FUNCTION "CENTR. 3  POSTERIORE DX" : VOID
TITLE =
VERSION : 0.1

BEGIN
NETWORK
TITLE =LETTURA STATUS WORD DA DRIVE
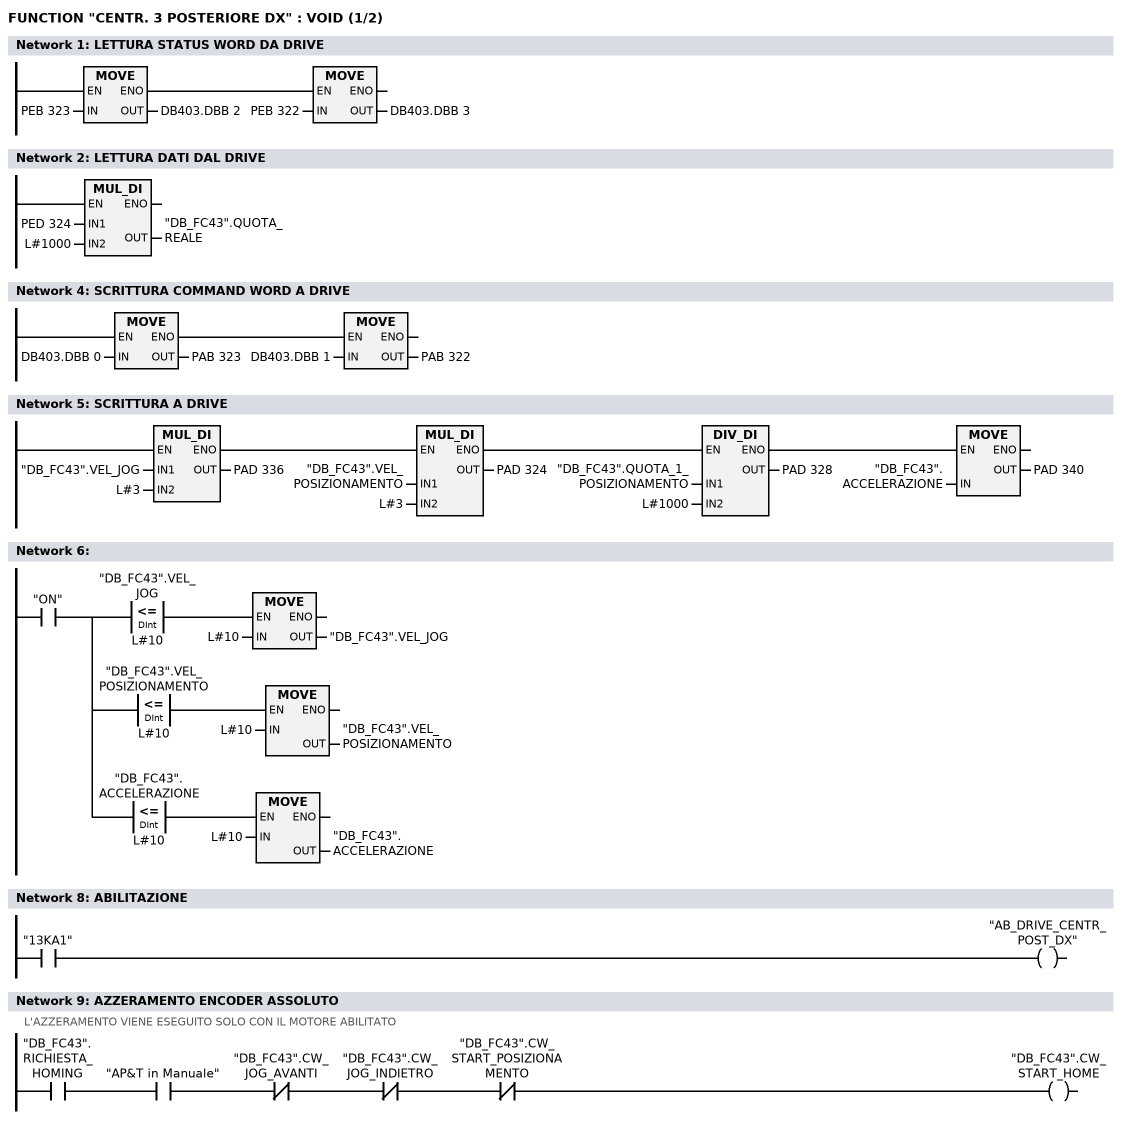
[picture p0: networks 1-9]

      U(    ;
      L     PEB  323;
      T     DB403.DBB    2;
      SET   ;
      SAVE  ;
      CLR   ;
      U     BIE;
      )     ;
      SPBNB _001;
      L     PEB  322;
      T     DB403.DBB    3;
_001: NOP   0;
NETWORK
TITLE =LETTURA DATI DAL DRIVE

      L     PED  324;
      L     L#1000;
      *D    ;
      T     "DB_FC43".QUOTA_REALE;
      NOP   0;
NETWORK
TITLE =

NETWORK
TITLE =SCRITTURA COMMAND WORD A DRIVE

      U(    ;
      L     DB403.DBB    0;
      T     PAB  323;
      SET   ;
      SAVE  ;
      CLR   ;
      U     BIE;
      )     ;
      SPBNB _002;
      L     DB403.DBB    1;
      T     PAB  322;
_002: NOP   0;
NETWORK
TITLE =SCRITTURA A DRIVE

      U(    ;
      U(    ;
      U(    ;
      L     "DB_FC43".VEL_JOG;
      L     L#3;
      *D    ;
      T     PAD  336;
      UN    OV;
      SAVE  ;
      CLR   ;
      U     BIE;
      )     ;
      SPBNB _003;
      L     "DB_FC43".VEL_POSIZIONAMENTO;
      L     L#3;
      *D    ;
      T     PAD  324;
      UN    OV;
      SAVE  ;
      CLR   ;
_003: U     BIE;
      )     ;
      SPBNB _004;
      L     "DB_FC43".QUOTA_1_POSIZIONAMENTO;
      L     L#1000;
      /D    ;
      T     PAD  328;
      UN    OV;
      SAVE  ;
      CLR   ;
_004: U     BIE;
      )     ;
      SPBNB _005;
      L     "DB_FC43".ACCELERAZIONE;
      T     PAD  340;
_005: NOP   0;
NETWORK
TITLE =

      U     "ON";
      =     L      0.0;
      U     L      0.0;
      U(    ;
      L     "DB_FC43".VEL_JOG;
      L     L#10;
      <=D   ;
      )     ;
      SPBNB _006;
      L     L#10;
      T     "DB_FC43".VEL_JOG;
_006: NOP   0;
      U     L      0.0;
      U(    ;
      L     "DB_FC43".VEL_POSIZIONAMENTO;
      L     L#10;
      <=D   ;
      )     ;
      SPBNB _007;
      L     L#10;
      T     "DB_FC43".VEL_POSIZIONAMENTO;
_007: NOP   0;
      U     L      0.0;
      U(    ;
      L     "DB_FC43".ACCELERAZIONE;
      L     L#10;
      <=D   ;
      )     ;
      SPBNB _008;
      L     L#10;
      T     "DB_FC43".ACCELERAZIONE;
_008: NOP   0;
NETWORK
TITLE =

NETWORK
TITLE =ABILITAZIONE

      U     "13KA1";
      =     "AB_DRIVE_CENTR_POST_DX";
NETWORK
TITLE =AZZERAMENTO ENCODER ASSOLUTO
//L'AZZERAMENTO VIENE ESEGUITO SOLO CON IL MOTORE ABILITATO
      U     "DB_FC43".RICHIESTA_HOMING;
      U     "AP&T in Manuale";
      UN    "DB_FC43".CW_JOG_AVANTI;
      UN    "DB_FC43".CW_JOG_INDIETRO;
      UN    "DB_FC43".CW_START_POSIZIONAMENTO;
      =     "DB_FC43".CW_START_HOME;
NETWORK
TITLE =COMANDI DI JOG
//N.B. VERIFICARE QUOTE EXTRACORSA SOFTWARE
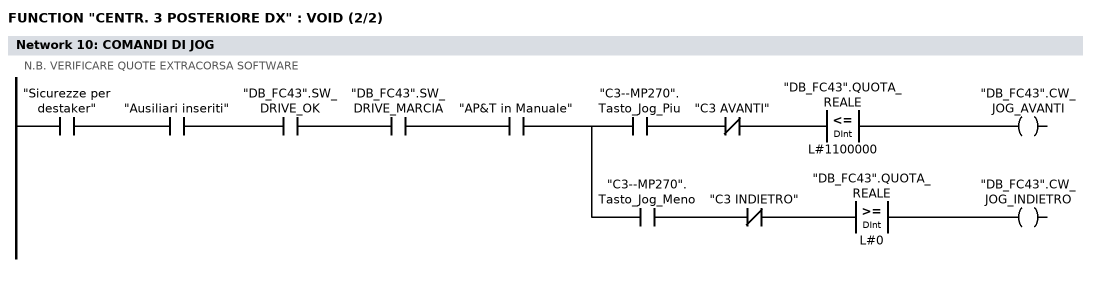
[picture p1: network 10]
      U     "Sicurezze per destaker";
      U     "Ausiliari inseriti";
      U     "DB_FC43".SW_DRIVE_OK;
      U     "DB_FC43".SW_DRIVE_MARCIA;
      U     "AP&T in Manuale";
      =     L      0.0;
      U     L      0.0;
      U     "C3--MP270".Tasto_Jog_Piu;
      UN    "C3 AVANTI";
      U(    ;
      L     "DB_FC43".QUOTA_REALE;
      L     L#1100000;
      <=D   ;
      )     ;
      =     "DB_FC43".CW_JOG_AVANTI;
      U     L      0.0;
      U     "C3--MP270".Tasto_Jog_Meno;
      UN    "C3 INDIETRO";
      U(    ;
      L     "DB_FC43".QUOTA_REALE;
      L     L#0;
      >=D   ;
      )     ;
      =     "DB_FC43".CW_JOG_INDIETRO;
NETWORK
TITLE =Centratore 3: Posizioni

      U     "ON";
      =     L      0.0;
      U     L      0.0;
      U(    ;
      L     "DB_FC43".QUOTA_REALE;
      L     L#100;
      <=D   ;
      )     ;
      U(    ;
      L     "DB_FC43".QUOTA_REALE;
      L     L#-100;
      >=D   ;
      )     ;
      =     "C3: Asse in pos.0";
      U(    ;
      U(    ;
      U     L      0.0;
      SPBNB _009;
      L     "MATRICOLA ATTUALE".C3_Posizione_1;
      L     L#100;
      -D    ;
      T     "CONFRONTI CENTRATORI".C3_Pos_1_Min;
      UN    OV;
      SAVE  ;
      CLR   ;
_009: U     BIE;
      )     ;
      SPBNB _00a;
      L     "MATRICOLA ATTUALE".C3_Posizione_1;
      L     L#200;
      +D    ;
      T     "CONFRONTI CENTRATORI".C3_Pos_1_Max;
      UN    OV;
      SAVE  ;
      CLR   ;
_00a: U     BIE;
      )     ;
      U(    ;
      L     "DB_FC43".QUOTA_REALE;
      L     "CONFRONTI CENTRATORI".C3_Pos_1_Min;
      >=D   ;
      )     ;
      U(    ;
      L     "DB_FC43".QUOTA_REALE;
      L     "CONFRONTI CENTRATORI".C3_Pos_1_Max;
      <=D   ;
      )     ;
      =     "C3: Asse in pos.1";
      U(    ;
      U(    ;
      U     L      0.0;
      SPBNB _00b;
      L     "MATRICOLA ATTUALE".C3_Posizione_2;
      L     L#100;
      -D    ;
      T     "CONFRONTI CENTRATORI".C3_Pos_2_Min;
      UN    OV;
      SAVE  ;
      CLR   ;
_00b: U     BIE;
      )     ;
      SPBNB _00c;
      L     "MATRICOLA ATTUALE".C3_Posizione_2;
      L     L#50000;
      +D    ;
      T     "CONFRONTI CENTRATORI".C3_Pos_2_Max;
      UN    OV;
      SAVE  ;
      CLR   ;
_00c: U     BIE;
      )     ;
      U(    ;
      L     "DB_FC43".QUOTA_REALE;
      L     "CONFRONTI CENTRATORI".C3_Pos_2_Min;
      >=D   ;
      )     ;
      UN    "C3: Asse in pos.3";
      UN    "C3: Asse in pos.4";
      =     "C3: Asse in pos.2";
      U(    ;
      U(    ;
      U     L      0.0;
      SPBNB _00d;
      L     "MATRICOLA ATTUALE".C3_Posizione_3;
      L     L#100;
      -D    ;
      T     "CONFRONTI CENTRATORI".C3_Pos_3_Min;
      UN    OV;
      SAVE  ;
      CLR   ;
_00d: U     BIE;
      )     ;
      SPBNB _00e;
      L     "MATRICOLA ATTUALE".C3_Posizione_3;
      L     L#50000;
      +D    ;
      T     "CONFRONTI CENTRATORI".C3_Pos_3_Max;
      UN    OV;
      SAVE  ;
      CLR   ;
_00e: U     BIE;
      )     ;
      U(    ;
      L     "DB_FC43".QUOTA_REALE;
      L     "CONFRONTI CENTRATORI".C3_Pos_3_Min;
      >=D   ;
      )     ;
      UN    "C3: Asse in pos.4";
      =     "C3: Asse in pos.3";
      U(    ;
      U(    ;
      U     L      0.0;
      SPBNB _00f;
      L     "MATRICOLA ATTUALE".C3_Posizione_4;
      L     L#100;
      -D    ;
      T     "CONFRONTI CENTRATORI".C3_Pos_4_Min;
      UN    OV;
      SAVE  ;
      CLR   ;
_00f: U     BIE;
      )     ;
      SPBNB _010;
      L     "MATRICOLA ATTUALE".C3_Posizione_4;
      L     L#100;
      +D    ;
      T     "CONFRONTI CENTRATORI".C3_Pos_4_Max;
      UN    OV;
      SAVE  ;
      CLR   ;
_010: U     BIE;
      )     ;
      U(    ;
      L     "DB_FC43".QUOTA_REALE;
      L     "CONFRONTI CENTRATORI".C3_Pos_4_Min;
      >=D   ;
      )     ;
      U(    ;
      L     "DB_FC43".QUOTA_REALE;
      L     "CONFRONTI CENTRATORI".C3_Pos_4_Max;
      <=D   ;
      )     ;
      =     "C3: Asse in pos.4";
NETWORK
TITLE =Centratore 3: consenso abilitazione
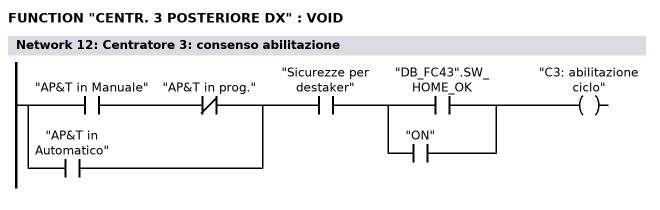
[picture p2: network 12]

      U(    ;
      U     "AP&T in Manuale";
      UN    "AP&T in prog.";
      O     "AP&T in Automatico";
      )     ;
      U     "Sicurezze per destaker";
      U(    ;
      O     "DB_FC43".SW_HOME_OK;
      O     "ON";
      )     ;
      =     "C3: abilitazione ciclo";
NETWORK
TITLE =Centratore 3: comando avvicinamento  (centraggi aperti)

      U(    ;
      U(    ;
      O     "Comando apre centraggi";
      O     "C3--MP270".Tasto_Indietro;
      O     ;
      U     "Apertura centratori";
      U(    ;
      O     "Centratori a riposo";
      O     "Centratori tutti chiusi";
      )     ;
      )     ;
      UN    "C3: Asse in pos.1";
      UN    "C3: comando arrivo";
      UN    "C3: comando a riposo";
      U     "C3: abilitazione ciclo";
      L     S5T#100MS;
      SE    T    187;
      NOP   0;
      NOP   0;
      NOP   0;
      U     T    187;
      )     ;
      S     "C3: comando avvicinam";
      U(    ;
      O     "C3: Asse in pos.1";
      O(    ;
      U(    ;
      O     "Ripristino centratori";
      O     "Comando riposo centraggi";
      O     "C3--MP270".Tasto_Riposo;
      )     ;
      FP    "C3: one shot 1";
      )     ;
      )     ;
      R     "C3: comando avvicinam";
      NOP   0;
NETWORK
TITLE =Centratore 3: comando arrivo (centraggi chiusi)

      U(    ;
      U(    ;
      O     "Comando chiude centraggi";
      O     "C3--MP270".Tasto_Avanti;
      O     ;
      U     "Chiusura centratori";
      U(    ;
      O     "Centratori tutti aperti";
      O     "Centratori a riposo";
      )     ;
      )     ;
      UN    "C3: Asse in pos.4";
      UN    "C3: comando avvicinam";
      UN    "C3: comando a riposo";
      U     "C3: abilitazione ciclo";
      L     S5T#100MS;
      SE    T    188;
      NOP   0;
      NOP   0;
      NOP   0;
      U     T    188;
      )     ;
      S     "C3: comando arrivo";
      U(    ;
      O     "C3: Asse in pos.4";
      O(    ;
      U(    ;
      O     "Ripristino centratori";
      O     "Comando riposo centraggi";
      O     "C3--MP270".Tasto_Riposo;
      )     ;
      FP    "C3: one shot 2";
      )     ;
      )     ;
      R     "C3: comando arrivo";
      NOP   0;
NETWORK
TITLE =Centratore 3: comando automatico centraggi a riposo

      U(    ;
      U(    ;
      O     "Comando riposo centraggi";
      O     "C3--MP270".Tasto_Riposo;
      )     ;
      UN    "C3: Asse in pos.0";
      UN    "C3: comando avvicinam";
      UN    "C3: comando arrivo";
      U     "C3: abilitazione ciclo";
      L     S5T#100MS;
      SE    T    189;
      NOP   0;
      NOP   0;
      NOP   0;
      U     T    189;
      )     ;
      S     "C3: comando a riposo";
      U(    ;
      O     "C3: Asse in pos.0";
      O(    ;
      U     "Ripristino centratori";
      FP    "C3: one shot 3";
      )     ;
      )     ;
      R     "C3: comando a riposo";
      NOP   0;
NETWORK
TITLE =Centratore 3: quote impostate per posizioni

      U     "ON";
      =     L      0.0;
      U(    ;
      U(    ;
      U     L      0.0;
      U     "C3: comando a riposo";
      UN    "C3: Asse in pos.0";
      SPBNB _011;
      L     0;
      T     "DB_FC43".QUOTA_1_POSIZIONAMENTO;
      SET   ;
      SAVE  ;
      CLR   ;
_011: U     BIE;
      )     ;
      SPBNB _012;
      L     L#150;
      T     "DB_FC43".VEL_POSIZIONAMENTO;
      SET   ;
      SAVE  ;
      CLR   ;
_012: U     BIE;
      )     ;
      SPBNB _013;
      L     L#1000;
      T     "DB_FC43".ACCELERAZIONE;
      SET   ;
      SAVE  ;
      CLR   ;
_013: U     BIE;
      =     "C3: Quote pronte pos.0";
      U(    ;
      U(    ;
      U     L      0.0;
      U     "C3: comando avvicinam";
      UN    "C3: Asse in pos.1";
      SPBNB _014;
      L     "MATRICOLA ATTUALE".C3_Posizione_1;
      T     "DB_FC43".QUOTA_1_POSIZIONAMENTO;
      SET   ;
      SAVE  ;
      CLR   ;
_014: U     BIE;
      )     ;
      SPBNB _015;
      L     "MATRICOLA ATTUALE".C3_Velocita_1;
      T     "DB_FC43".VEL_POSIZIONAMENTO;
      SET   ;
      SAVE  ;
      CLR   ;
_015: U     BIE;
      )     ;
      SPBNB _016;
      L     "MATRICOLA ATTUALE".C3_Accell_1;
      T     "DB_FC43".ACCELERAZIONE;
      SET   ;
      SAVE  ;
      CLR   ;
_016: U     BIE;
      =     "C3: Quote pronte pos.1";
      U     L      0.0;
      U     "C3: comando arrivo";
      =     L      0.1;
      U(    ;
      U(    ;
      U     L      0.1;
      UN    "C3: Asse in pos.2";
      SPBNB _017;
      L     "MATRICOLA ATTUALE".C3_Posizione_4;
      T     "DB_FC43".QUOTA_1_POSIZIONAMENTO;
      SET   ;
      SAVE  ;
      CLR   ;
_017: U     BIE;
      )     ;
      SPBNB _018;
      L     "MATRICOLA ATTUALE".C3_Velocita_2;
      T     "DB_FC43".VEL_POSIZIONAMENTO;
      SET   ;
      SAVE  ;
      CLR   ;
_018: U     BIE;
      )     ;
      SPBNB _019;
      L     "MATRICOLA ATTUALE".C3_Accell_2;
      T     "DB_FC43".ACCELERAZIONE;
      SET   ;
      SAVE  ;
      CLR   ;
_019: U     BIE;
      S     "C3: Quote pronte pos.2";
      U     L      0.1;
      U     "C3: Quote pronte pos.2";
      UN    "C3: Reset start pos.2";
      L     S5T#1S;
      SE    "C3: ritardo P2";
      NOP   0;
      NOP   0;
      NOP   0;
      U     "C3: ritardo P2";
      S     "C3: Reset start pos.2";
      R     "C3: Quote pronte pos.2";
      U     L      0.0;
      U     "C3: comando arrivo";
      =     L      0.1;
      U(    ;
      U(    ;
      U(    ;
      U     L      0.1;
      U     "C3: Asse in pos.2";
      UN    "C3: Asse in pos.3";
      SPBNB _01a;
      L     "MATRICOLA ATTUALE".C3_Posizione_4;
      T     "DB_FC43".QUOTA_1_POSIZIONAMENTO;
      SET   ;
      SAVE  ;
      CLR   ;
_01a: U     BIE;
      )     ;
      SPBNB _01b;
      L     "MATRICOLA ATTUALE".C3_Velocita_3;
      T     "DB_FC43".VEL_POSIZIONAMENTO;
      SET   ;
      SAVE  ;
      CLR   ;
_01b: U     BIE;
      )     ;
      SPBNB _01c;
      L     "MATRICOLA ATTUALE".C3_Accell_3;
      T     "DB_FC43".ACCELERAZIONE;
      SET   ;
      SAVE  ;
      CLR   ;
_01c: U     BIE;
      )     ;
      U     "C3: Reset start pos.2";
      S     "C3: Quote pronte pos.3";
      R     "C3: Reset start pos.2";
      U     L      0.1;
      U     "C3: Quote pronte pos.3";
      L     S5T#500MS;
      SE    "C3: ritardo P3";
      NOP   0;
      NOP   0;
      NOP   0;
      U     "C3: ritardo P3";
      S     "C3: Reset start pos.3";
      R     "C3: Quote pronte pos.3";
      U     L      0.0;
      U     "C3: comando arrivo";
      =     L      0.1;
      U(    ;
      U(    ;
      U(    ;
      U     L      0.1;
      U     "C3: Asse in pos.3";
      UN    "C3: Asse in pos.4";
      SPBNB _01d;
      L     "MATRICOLA ATTUALE".C3_Posizione_4;
      T     "DB_FC43".QUOTA_1_POSIZIONAMENTO;
      SET   ;
      SAVE  ;
      CLR   ;
_01d: U     BIE;
      )     ;
      SPBNB _01e;
      L     "MATRICOLA ATTUALE".C3_Velocita_4;
      T     "DB_FC43".VEL_POSIZIONAMENTO;
      SET   ;
      SAVE  ;
      CLR   ;
_01e: U     BIE;
      )     ;
      SPBNB _01f;
      L     "MATRICOLA ATTUALE".C3_Accell_4;
      T     "DB_FC43".ACCELERAZIONE;
      SET   ;
      SAVE  ;
      CLR   ;
_01f: U     BIE;
      )     ;
      U     "C3: Reset start pos.3";
      S     "C3: Quote pronte pos.4";
      R     "C3: Reset start pos.3";
      U     L      0.1;
      U     "C3: Quote pronte pos.4";
      L     S5T#500MS;
      SE    "C3: ritardo P4";
      NOP   0;
      NOP   0;
      NOP   0;
      U     "C3: ritardo P4";
      S     "C3: Reset start pos.4";
      R     "C3: Quote pronte pos.4";
NETWORK
TITLE =Centratore 3: reset impostate
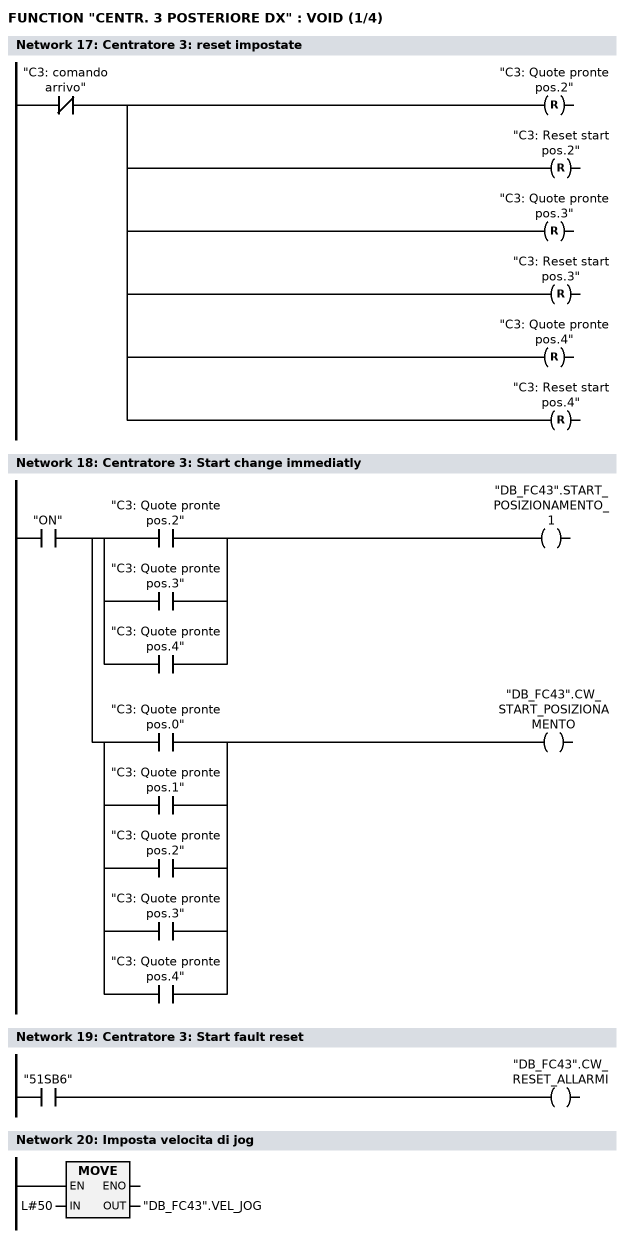
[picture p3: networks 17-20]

      UN    "C3: comando arrivo";
      R     "C3: Quote pronte pos.2";
      R     "C3: Reset start pos.2";
      R     "C3: Quote pronte pos.3";
      R     "C3: Reset start pos.3";
      R     "C3: Quote pronte pos.4";
      R     "C3: Reset start pos.4";
NETWORK
TITLE =Centratore 3: Start change immediatly

      U     "ON";
      =     L      0.0;
      U     L      0.0;
      U(    ;
      O     "C3: Quote pronte pos.2";
      O     "C3: Quote pronte pos.3";
      O     "C3: Quote pronte pos.4";
      )     ;
      =     "DB_FC43".START_POSIZIONAMENTO_1;
      U     L      0.0;
      U(    ;
      O     "C3: Quote pronte pos.0";
      O     "C3: Quote pronte pos.1";
      O     "C3: Quote pronte pos.2";
      O     "C3: Quote pronte pos.3";
      O     "C3: Quote pronte pos.4";
      )     ;
      =     "DB_FC43".CW_START_POSIZIONAMENTO;
NETWORK
TITLE =Centratore 3: Start fault reset

      U     "51SB6";
      =     "DB_FC43".CW_RESET_ALLARMI;
NETWORK
TITLE =Imposta velocita di jog

      L     L#50;
      T     "DB_FC43".VEL_JOG;
      NOP   0;
NETWORK
TITLE =Centratore 1: Drive Enable ok
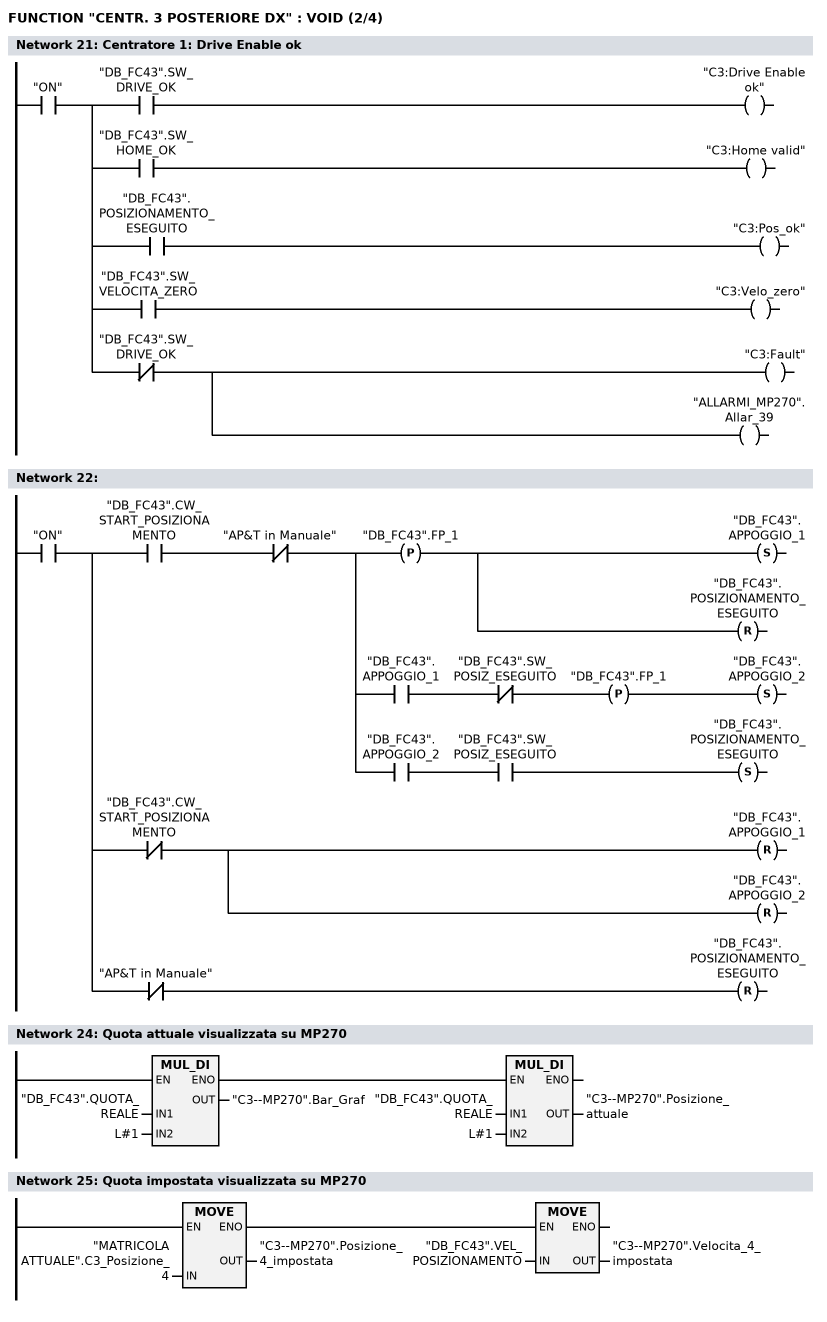
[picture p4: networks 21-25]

      U     "ON";
      =     L      0.0;
      U     L      0.0;
      U     "DB_FC43".SW_DRIVE_OK;
      =     "C3:Drive Enable ok";
      U     L      0.0;
      U     "DB_FC43".SW_HOME_OK;
      =     "C3:Home valid";
      U     L      0.0;
      U     "DB_FC43".POSIZIONAMENTO_ESEGUITO;
      =     "C3:Pos_ok";
      U     L      0.0;
      U     "DB_FC43".SW_VELOCITA_ZERO;
      =     "C3:Velo_zero";
      U     L      0.0;
      UN    "DB_FC43".SW_DRIVE_OK;
      =     "C3:Fault";
      =     "ALLARMI_MP270".Allar_39;
NETWORK
TITLE =

      U     "ON";
      =     L      0.0;
      U     L      0.0;
      U     "DB_FC43".CW_START_POSIZIONAMENTO;
      UN    "AP&T in Manuale";
      =     L      0.1;
      U     L      0.1;
      FP    "DB_FC43".FP_1;
      S     "DB_FC43".APPOGGIO_1;
      R     "DB_FC43".POSIZIONAMENTO_ESEGUITO;
      U     L      0.1;
      U     "DB_FC43".APPOGGIO_1;
      UN    "DB_FC43".SW_POSIZ_ESEGUITO;
      FP    "DB_FC43".FP_1;
      S     "DB_FC43".APPOGGIO_2;
      U     L      0.1;
      U     "DB_FC43".APPOGGIO_2;
      U     "DB_FC43".SW_POSIZ_ESEGUITO;
      S     "DB_FC43".POSIZIONAMENTO_ESEGUITO;
      U     L      0.0;
      UN    "DB_FC43".CW_START_POSIZIONAMENTO;
      R     "DB_FC43".APPOGGIO_1;
      R     "DB_FC43".APPOGGIO_2;
      U     L      0.0;
      UN    "AP&T in Manuale";
      R     "DB_FC43".POSIZIONAMENTO_ESEGUITO;
NETWORK
TITLE =

NETWORK
TITLE =Quota attuale visualizzata su MP270

      U(    ;
      L     "DB_FC43".QUOTA_REALE;
      L     L#1;
      *D    ;
      T     "C3--MP270".Bar_Graf;
      UN    OV;
      SAVE  ;
      CLR   ;
      U     BIE;
      )     ;
      SPBNB _020;
      L     "DB_FC43".QUOTA_REALE;
      L     L#1;
      *D    ;
      T     "C3--MP270".Posizione_attuale;
_020: NOP   0;
NETWORK
TITLE =Quota impostata visualizzata su MP270

      U(    ;
      L     "MATRICOLA ATTUALE".C3_Posizione_4;
      T     "C3--MP270".Posizione_4_impostata;
      SET   ;
      SAVE  ;
      CLR   ;
      U     BIE;
      )     ;
      SPBNB _021;
      L     "DB_FC43".VEL_POSIZIONAMENTO;
      T     "C3--MP270".Velocita_4_impostata;
_021: NOP   0;
NETWORK
TITLE =Visualizza FC su MP270
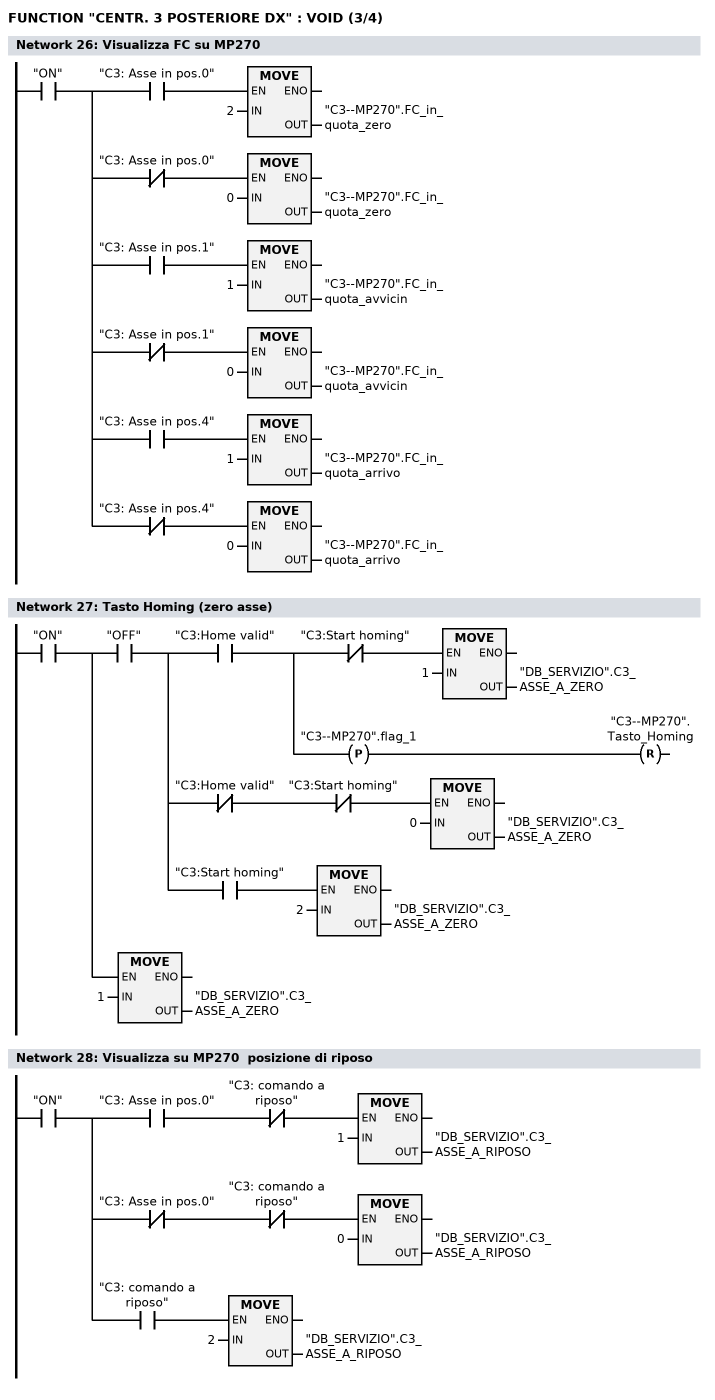
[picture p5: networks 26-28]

      U     "ON";
      =     L      0.0;
      U     L      0.0;
      U     "C3: Asse in pos.0";
      SPBNB _022;
      L     2;
      T     "C3--MP270".FC_in_quota_zero;
_022: NOP   0;
      U     L      0.0;
      UN    "C3: Asse in pos.0";
      SPBNB _023;
      L     0;
      T     "C3--MP270".FC_in_quota_zero;
_023: NOP   0;
      U     L      0.0;
      U     "C3: Asse in pos.1";
      SPBNB _024;
      L     1;
      T     "C3--MP270".FC_in_quota_avvicin;
_024: NOP   0;
      U     L      0.0;
      UN    "C3: Asse in pos.1";
      SPBNB _025;
      L     0;
      T     "C3--MP270".FC_in_quota_avvicin;
_025: NOP   0;
      U     L      0.0;
      U     "C3: Asse in pos.4";
      SPBNB _026;
      L     1;
      T     "C3--MP270".FC_in_quota_arrivo;
_026: NOP   0;
      U     L      0.0;
      UN    "C3: Asse in pos.4";
      SPBNB _027;
      L     0;
      T     "C3--MP270".FC_in_quota_arrivo;
_027: NOP   0;
NETWORK
TITLE =Tasto Homing (zero asse)

      U     "ON";
      =     L      0.0;
      U     L      0.0;
      U     "OFF";
      =     L      0.1;
      U     L      0.1;
      U     "C3:Home valid";
      =     L      0.2;
      U     L      0.2;
      UN    "C3:Start homing";
      SPBNB _028;
      L     1;
      T     "DB_SERVIZIO".C3_ASSE_A_ZERO;
_028: NOP   0;
      U     L      0.2;
      FP    "C3--MP270".flag_1;
      R     "C3--MP270".Tasto_Homing;
      U     L      0.1;
      UN    "C3:Home valid";
      UN    "C3:Start homing";
      SPBNB _029;
      L     0;
      T     "DB_SERVIZIO".C3_ASSE_A_ZERO;
_029: NOP   0;
      U     L      0.1;
      U     "C3:Start homing";
      SPBNB _02a;
      L     2;
      T     "DB_SERVIZIO".C3_ASSE_A_ZERO;
_02a: NOP   0;
      U     L      0.0;
      SPBNB _02b;
      L     1;
      T     "DB_SERVIZIO".C3_ASSE_A_ZERO;
_02b: NOP   0;
NETWORK
TITLE =Visualizza su MP270  posizione di riposo

      U     "ON";
      =     L      0.0;
      U     L      0.0;
      U     "C3: Asse in pos.0";
      UN    "C3: comando a riposo";
      SPBNB _02c;
      L     1;
      T     "DB_SERVIZIO".C3_ASSE_A_RIPOSO;
_02c: NOP   0;
      U     L      0.0;
      UN    "C3: Asse in pos.0";
      UN    "C3: comando a riposo";
      SPBNB _02d;
      L     0;
      T     "DB_SERVIZIO".C3_ASSE_A_RIPOSO;
_02d: NOP   0;
      U     L      0.0;
      U     "C3: comando a riposo";
      SPBNB _02e;
      L     2;
      T     "DB_SERVIZIO".C3_ASSE_A_RIPOSO;
_02e: NOP   0;
NETWORK
TITLE =Visualizza su MP270  posizione di avvicinamento
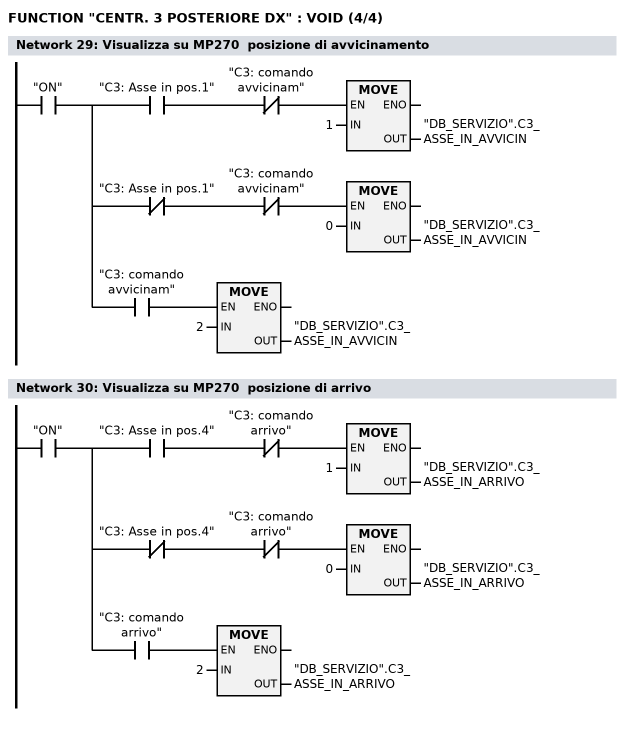
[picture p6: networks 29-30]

      U     "ON";
      =     L      0.0;
      U     L      0.0;
      U     "C3: Asse in pos.1";
      UN    "C3: comando avvicinam";
      SPBNB _02f;
      L     1;
      T     "DB_SERVIZIO".C3_ASSE_IN_AVVICIN;
_02f: NOP   0;
      U     L      0.0;
      UN    "C3: Asse in pos.1";
      UN    "C3: comando avvicinam";
      SPBNB _030;
      L     0;
      T     "DB_SERVIZIO".C3_ASSE_IN_AVVICIN;
_030: NOP   0;
      U     L      0.0;
      U     "C3: comando avvicinam";
      SPBNB _031;
      L     2;
      T     "DB_SERVIZIO".C3_ASSE_IN_AVVICIN;
_031: NOP   0;
NETWORK
TITLE =Visualizza su MP270  posizione di arrivo

      U     "ON";
      =     L      0.0;
      U     L      0.0;
      U     "C3: Asse in pos.4";
      UN    "C3: comando arrivo";
      SPBNB _032;
      L     1;
      T     "DB_SERVIZIO".C3_ASSE_IN_ARRIVO;
_032: NOP   0;
      U     L      0.0;
      UN    "C3: Asse in pos.4";
      UN    "C3: comando arrivo";
      SPBNB _033;
      L     0;
      T     "DB_SERVIZIO".C3_ASSE_IN_ARRIVO;
_033: NOP   0;
      U     L      0.0;
      U     "C3: comando arrivo";
      SPBNB _034;
      L     2;
      T     "DB_SERVIZIO".C3_ASSE_IN_ARRIVO;
_034: NOP   0;
END_FUNCTION

